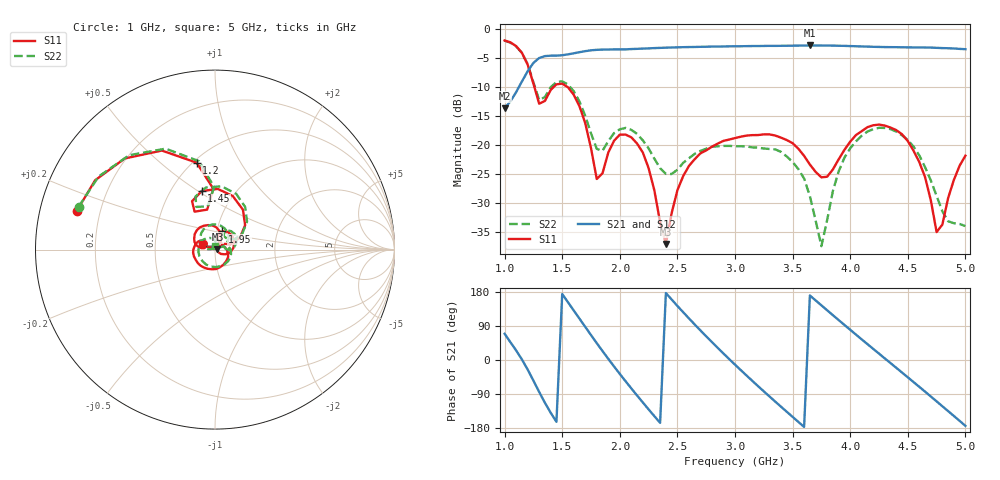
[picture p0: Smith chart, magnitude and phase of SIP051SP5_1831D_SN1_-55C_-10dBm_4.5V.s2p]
# GHz  S  dB  R  50
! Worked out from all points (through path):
!   81 points, 1 GHz to 5 GHz, reference 50 ohm
!   highest |S21| = -2.80 dB at 3.65 GHz (marker M1); lowest = -13.7 dB at 1 GHz (marker M2)
!   lowest |S11| = -37.1 dB at 2.4 GHz (marker M3), VSWR 1.03, Z = 51.4 + j0.151 ohm
!   |S11| at or under -10 dB: 1.259 GHz to 1.426 GHz (166.9 MHz wide, 12.4 % of centre); 1.547 GHz to end of sweep
!   |S22| runs from -37.5 to -2.0 dB; largest |S21 - S12| = 0.002
!   S11 on the Smith chart (normalised r, x): 1 GHz: 0.11, +0.13; 1.2 GHz: 0.52, +0.67; 1.45 GHz: 0.71, +0.52; 1.95 GHz: 1.06, +0.22; 5 GHz: 0.86, +0.06
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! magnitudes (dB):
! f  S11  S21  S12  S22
! 1 GHz  -1.9  -13.7  -13.7  -2.0
! 1.2 GHz  -6.1  -7.3  -7.3  -6.0
! 1.3 GHz  -12.9  -5.0  -5.0  -12.2
! 1.45 GHz  -9.5  -4.6  -4.5  -9.1
! 1.7 GHz  -16.2  -3.8  -3.8  -15.0
! 1.8 GHz  -25.9  -3.6  -3.6  -20.7
! 1.95 GHz  -19.3  -3.5  -3.5  -18.0
! 2.2 GHz  -21.3  -3.3  -3.3  -19.2
! 2.35 GHz  -33.4  -3.2  -3.2  -24.0
! 2.4 GHz  -37.1  -3.2  -3.2  -25.0
! 2.5 GHz  -27.9  -3.1  -3.1  -24.3
! 2.6 GHz  -23.6  -3.1  -3.1  -22.3
! 3 GHz  -18.8  -2.9  -2.9  -20.2
! 3.4 GHz  -18.8  -2.9  -2.9  -21.2
! 3.65 GHz  -23.4  -2.8  -2.8  -28.9
! 3.7 GHz  -24.7  -2.8  -2.8  -33.1
! 3.75 GHz  -25.6  -2.8  -2.8  -37.5
! 3.95 GHz  -20.9  -2.9  -2.9  -22.2
! 4.35 GHz  -17.0  -3.1  -3.1  -17.3
! 4.6 GHz  -23.0  -3.1  -3.1  -21.8
! 4.75 GHz  -35.1  -3.2  -3.2  -28.8
! 5 GHz  -21.9  -3.4  -3.5  -34.0
